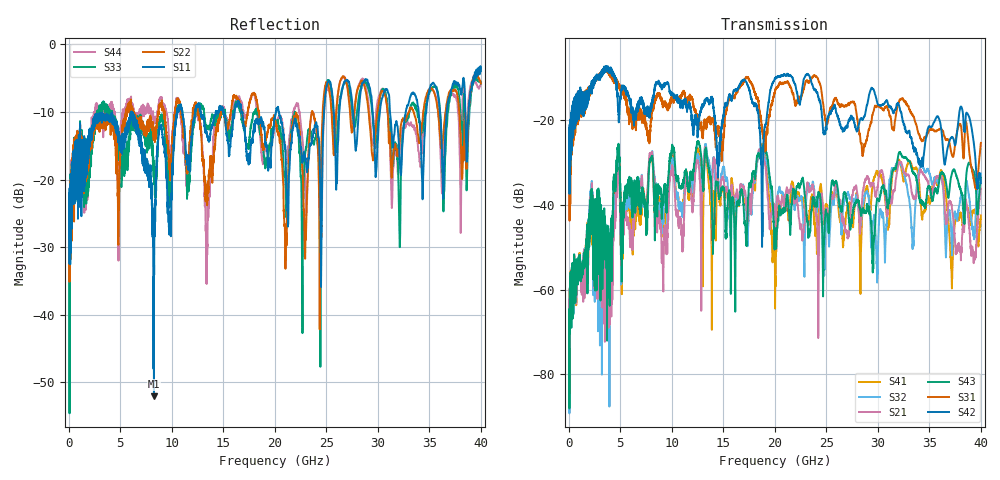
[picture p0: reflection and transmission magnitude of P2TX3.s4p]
!Agilent Technologies,N5245A,MY49151084,A.09.20.08
!Agilent N5245A: A.09.20.08
!Date: Thursday, March 01, 2012 12:02:11
!Correction: S11(Full 4 Port(1,2,3,4))
!S12(Full 4 Port(1,2,3,4))
!S13(Full 4 Port(1,2,3,4))
!S14(Full 4 Port(1,2,3,4))
!S21(Full 4 Port(1,2,3,4))
!S22(Full 4 Port(1,2,3,4))
!S23(Full 4 Port(1,2,3,4))
!S24(Full 4 Port(1,2,3,4))
!S31(Full 4 Port(1,2,3,4))
!S32(Full 4 Port(1,2,3,4))
!S33(Full 4 Port(1,2,3,4))
!S34(Full 4 Port(1,2,3,4))
!S41(Full 4 Port(1,2,3,4))
!S42(Full 4 Port(1,2,3,4))
!S43(Full 4 Port(1,2,3,4))
!S44(Full 4 Port(1,2,3,4))
!S4P File: Measurements: <S11,S12,S13,S14>,
!<S21,S22,S23,S24>,
!<S31,S32,S33,S34>,
!<S41,S42,S43,S44>:
# Hz S  dB  R 50
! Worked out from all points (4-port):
!   3996 points, 50 MHz to 40 GHz, reference 50 ohm
!   strongest paths, dB at 50 MHz, 10.04 GHz, 20.03 GHz, 30.02 GHz, 40 GHz:
!     S42: -25.3, -13.9, -10.1, -16.2, -34.9
!     S31: -25.5, -15.2, -13.0, -16.6, -25.3
!     S43: -65.8, -26.0, -45.4, -38.6, -33.6
!     S21: -63.8, -31.0, -45.1, -35.2, -36.2
!     S32: -63.4, -29.2, -43.4, -50.2, -32.7
!     S41: -62.4, -28.0, -64.4, -32.8, -42.5
!   lowest |S11| = -52.1 dB at 8.28 GHz (marker M1), VSWR 1.00, Z = 49.9 + j0.227 ohm
!   |S11| at or under -10 dB: start of sweep to 6.099 GHz; 6.101 GHz to 10.55 GHz (4.444 GHz wide, 53.4 % of centre); 20.39 GHz to 24.78 GHz (4.387 GHz wide, 19.4 % of centre)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
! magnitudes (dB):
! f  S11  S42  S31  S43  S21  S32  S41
! 50 MHz  -24.0  -25.3  -25.5  -65.8  -63.8  -63.4  -62.4
! 2.2 GHz  -13.4  -12.9  -12.9  -38.4  -36.4  -35.9  -38.3
! 4.06 GHz  -10.8  -8.8  -9.4  -56.5  -52.0  -49.2  -64.5
! 4.77 GHz  -13.4  -15.4  -11.4  -26.4  -32.5  -30.7  -28.5
! 8.28 GHz  -52.1  -13.7  -16.4  -38.3  -32.2  -32.2  -37.8
! 9.17 GHz  -14.5  -12.0  -16.1  -39.0  -58.6  -44.5  -45.5
! 40 GHz  -4.0  -34.9  -25.3  -33.6  -36.2  -32.7  -42.5
